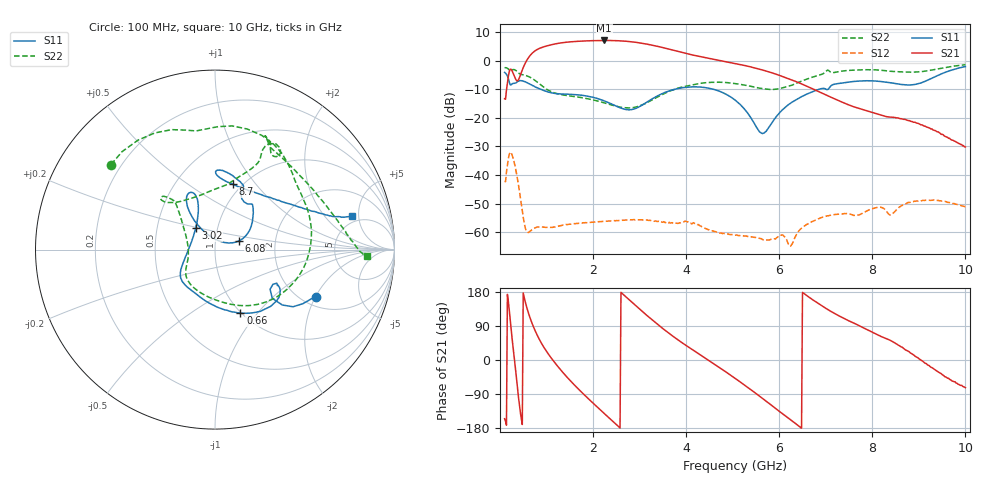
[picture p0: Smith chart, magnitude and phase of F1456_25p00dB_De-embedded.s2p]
! Integrated Device Technology
! Corporate Headquarters
! 6024 Silver Creek Valley Road
! San Jose, CA 95138  USA
! Phone:  1-408-284-8200
! Toll Free:  1-800-223-1366
! Webpage:  http://www.idt.com/
! Timing and RF Division
! 515 Groton Road, Suite 102
! Westford, MA 01886-6024
! Device:  F1456
! Description: 6-bit 0.5 dB Transmit Variable Gain Amplifier
! Frequency:  2100.0 -  2950.00 MHz
! Package:  6x6 mm Thin QFN Plastic Package: 28 pin
! State:  50
! Atten State:  25.0 dB
! Voltage:  +5.00 Volts
! Current:  216.965 mA
! Data:  The device was measured on a the F1455 evaluation board which has
!  individual transmission lines to the RF pins.  Data was collected
!  using a calibrated network analyzer.  The evaluation board was
!  de-embedded using a TRL calibration technique.
!  The reference plane is the edge of the package pin.
!  Pin  1 = CSb
!  Pin  2 = DATA
!  Pin  3 = CLK
!  Pin  4 = RSET
!  Pin  5 = GND
!  Pin  6 = RFIN  = Port 1
!  Pin  7 = GND
!  Pin  8 = NC
!  Pin  9 = NC
!  Pin 10 = NC
!  Pin 11 = NC
!  Pin 12 = NC
!  Pin 13 = NC
!  Pin 14 = /STBY
!  Pin 15 = GND
!  Pin 16 = RFOUT  = Port 2
!  Pin 17 = GND
!  Pin 18 = NC
!  Pin 19 = NC
!  Pin 20 = NC
!  Pin 21 = GND
!  Pin 22 = NC
!  Pin 23 = GND
!  Pin 24 = NC
!  Pin 25 = NC
!  Pin 26 = NC
!  Pin 27 = GND
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# GHz S dB R 50
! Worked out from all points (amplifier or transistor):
!   496 points, 100 MHz to 10 GHz, reference 50 ohm
!   highest |S21| = 7.0 dB at 2.24 GHz (marker M1)
!   |S21| within 3 dB of that: 818.4 MHz to 3.625 GHz (2.806 GHz wide, 126 % of centre)
!   unconditionally stable (mu >= 1): start of sweep to end of sweep
!   at 1.74 GHz: K = 139.58, MAG = 7.3 dB, |S12| = -56.7 dB
!   at 5.06 GHz: K = 511.36, MAG = -0.1 dB, |S12| = -61.0 dB
!   at 10 GHz: K = 637.29, MAG = -20.6 dB, |S12| = -51.1 dB
!   S11 on the Smith chart (normalised r, x): 100 MHz: 2.37, -2.02; 660 MHz: 0.99, -0.82; 3.02 GHz: 0.78, +0.19; 6.08 GHz: 1.30, +0.13; 8.7 GHz: 0.91, +0.77; 10 GHz: 4.20, +4.08
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0.1  -4.13 -24.9  -13.34 -155.1  -42.29 50.1  -2.52 140.8
0.24  -8.49 -31.0  -3.06 81.0  -32.22 -76.9  -3.44 94.5
0.32  -7.93 -29.5  -5.88 -7.6  -36.53 -154.8  -3.25 67.8
0.42  -7.03 -36.8  -5.91 -121.1  -45.78 139.9  -4.61 40.7
0.54  -7.39 -53.7  -1.02 155.3  -58.24 127.5  -5.14 15.8
0.66  -8.40 -68.1  2.00 106.6  -59.48 144.9  -5.94 -11.5
0.84  -9.81 -86.8  4.20 55.8  -58.15 117.0  -8.01 -48.7
1.16  -11.41 -113.2  5.72 -4.2  -58.14 80.6  -11.24 -92.9
1.48  -11.78 -130.4  6.49 -50.4  -57.21 58.9  -12.32 -119.9
1.76  -12.12 -140.6  6.80 -85.7  -56.75 44.2  -12.97 -134.3
2.24  -14.08 -156.0  7.02 -141.1  -56.14 24.4  -14.77 -150.3
2.62  -16.74 178.1  6.85 176.3  -55.78 9.9  -16.38 -167.7
3.02  -15.88 132.2  6.14 132.2  -55.70 -8.3  -15.68 162.4
3.4  -12.23 112.3  4.91 92.7  -56.13 -24.7  -12.62 140.8
4.12  -9.21 113.1  2.01 28.5  -57.08 -58.4  -8.53 131.0
5.06  -13.91 125.3  -1.03 -49.1  -61.01 -107.3  -8.04 137.0
5.64  -25.50 69.0  -3.29 -101.3  -62.54 -155.6  -9.82 121.7
6.08  -17.06 19.8  -5.65 -142.8  -60.99 168.3  -9.50 90.8
6.7  -10.98 41.4  -9.75 160.6  -56.29 149.1  -5.87 65.0
8.36  -7.69 88.2  -19.72 53.3  -53.76 66.3  -3.71 62.5
8.7  -8.47 74.7  -20.52 27.8  -50.08 70.9  -4.01 51.2
10  -2.11 13.8  -30.19 -72.8  -51.11 -23.9  -1.46 -2.6
